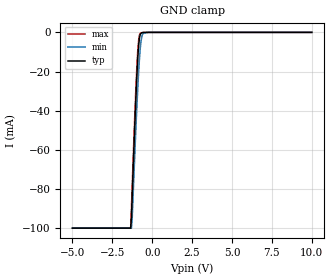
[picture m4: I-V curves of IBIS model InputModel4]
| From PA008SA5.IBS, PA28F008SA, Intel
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|**********************Input Model 4***************************************
[Model]   InputModel4
Model_type   Input
|   For RP#
Vinl = 0.8V
Vinh = 2.0V
| Variable   typ   min   max
C_comp   5.61p   NA   7.6p
[Voltage Range]   5.0V   4.5V   5.5V
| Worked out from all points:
|   GND clamp passes 1 mA (typ) near -0.74 V on its own axis
[GND_clamp]
|Voltage I(typ)   I(min)   I(max)
-5V       -99.86mA   -99.86mA   -99.85mA
-1.35V    -99.86mA   -99.86mA   -99.85mA
-1.3V     -94.35mA   -99.86mA   -88.84mA
-1.25V    -82.82mA   -94.23mA   -77.11mA
-1.1V     -49.42mA   -63.96mA   -43.91mA
-950mV    -20.26mA   -36.09mA   -15.49mA
-850mV    -6.695mA   -20.27mA   -3.804mA
-750mV    -1.086mA   -8.223mA   -522.9uA
-700mV    -433.8uA   -4.416mA   -274.8uA
-600mV    -126uA     -900.8uA   -99.63uA
-250mV    0A         0A         0A
10V       0A         0A         0A
[POWER_clamp]
| Input buffer circuits of this product do not intrinsically
| require a [POWER_clamp] definition.  This zero current
| [POWER_clamp] is provided for compatibility with some ibis
| parsers.
|   Voltage  I(typ)   I(min)   I(max)
-5V       0A         0A         0A
-4.75V    0A         0A         0A
9.75V     0A         0A         0A
10V       0A         0A         0A
